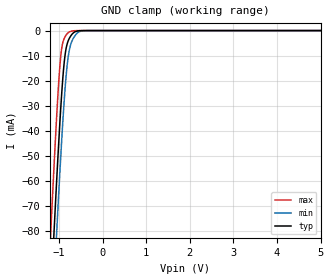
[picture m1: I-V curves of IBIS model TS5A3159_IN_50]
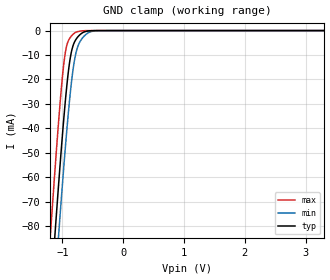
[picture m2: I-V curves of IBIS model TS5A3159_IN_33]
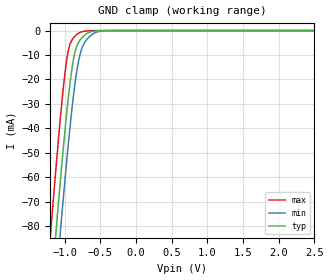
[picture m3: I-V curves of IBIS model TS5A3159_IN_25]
| TEXAS INSTRUMENTS INCORPORATED
| Standard Linear and Logic Group
| IBIS Model of TS5A3159
| 1-OHM SPDT ANALOG SWITCH
| This file contains package information for the following:
|  SOT 6-pin (DBV) package as [Component] TS5A3159_DBV
| This device can be powered at the following Vccs:
|  5 volt Vcc
|  3.3 volt Vcc
|  2.5 volt Vcc
|  1.8 volt Vcc
| This file provides unique models under the [Model Selector] for each Vcc.
| For operation at a specific Vcc, select the appropriate model after each
| [Model Selector] keyword.
[IBIS Ver]   3.2
[Comment char]  |_char
[File Name]   ts5a3159.ibs
[File Rev]   1.1 | a_die
[Date]   January 6, 2009
[Source]   Data created from TI-SPICE simulations at TI-SLL.
[Notes]   The following is an IBIS list for the TS5A3159.
   Please contact sllibis@ti.com with questions and
   comments concerning SLL IBIS models.
   - FILE REV HISTORY
   - 1.1 Release IBIS file on 01/08/09.
   - Power clamp data deleted was deleted as there is no
   power-clamp diode.
   - Non-monotonic data due to FET characteristics.
[Disclaimer] Property of Texas Instruments Incorporated.  Unauthorized
   reproduction and/or distribution is strictly prohibited.
   This product is protected under copyright law.
   Created  2009, (C) Copyright  2009, Texas Instruments
   Incorporated, All Rights Reserved
   UNLESS THERE IS A SIGNED, WRITTEN AGREEMENT TO THE
   CONTRARY, TEXAS INSTRUMENTS (TI) IS PROVIDING THE IBIS
   MODELS  AND WITHOUT ANY WARRANTY, EXPRESSED OR
   IMPLIED.  TI assumes no liability for:
   1) the accuracy of the IBIS models provided to your
   company;
   2) the proper functioning of these IBIS Models in your
   design or for any resulting applications; or
   3) infringement of patents, copyrights or intellectual
   property rights resulting from your use of these IBIS
   models.
   TI provides IBIS Models as a service to our customers.
   You and your company shall not distribute, sell or give
   these models to anyone else without prior written
   permission from TI.
   TI reserves the right to make changes to our products or
   to discontinue any semiconductor product or service
   without notice, and advises our customers to obtain the
   latest version of relevant information to verify, before
   placing orders, that the information being relied on is
   current.
   Please be aware that your receipt and use of the IBIS
   information provided shall serve as acceptance of these
   terms and conditions.  If you do not accept these terms,
   you should return or destroy the IBIS models and any
   other accompanying information immediately.
| Component TS5A3159_DBV 6-PIN SOT
[Component]   TS5A3159_DBV
[Manufacturer]   Texas Instruments, Inc.
[Package]
|   typ   min   max
R_pkg   2.500e-02   1.900e-02   3.700e-02
L_pkg   1.524e-09   1.260e-09   1.751e-09
C_pkg   2.450e-13   1.980e-13   2.640e-13
[Pin]   signal_name   model_name   R_pin   L_pin   C_pin
1   NO   TS5A3159_NX   2.100e-02   1.405e-09   2.460e-13
2   GND   GND   3.700e-02   1.751e-09   2.630e-13
3   NC   TS5A3159_NX   2.600e-02   1.493e-09   2.470e-13
4   COM   TS5A3159_COM   1.900e-02   1.620e-09   2.640e-13
5   VP   POWER   2.400e-02   1.260e-09   1.980e-13
6   IN   TS5A3159_IN   2.100e-02   1.617e-09   2.500e-13
[Series Switch Groups]
| Function Group States
On  1 /   | NO->COM IN HIGH
   | COM->NO IN HIGH
On  2 /   | NC->COM IN LOW
   | COM->NC IN LOW
On  1 /   | IN HIGH
[Series Pin Mapping]   pin_2   model_name   function_table_group
1   4   TS5A3159_NX_S   1
4   1   TS5A3159_COM_S   1
3   4   TS5A3159_NX_S   2
4   3   TS5A3159_COM_S   2
| Model TS5A3159_IN
[Model Selector]   TS5A3159_IN
TS5A3159_IN_50   5 volt Vcc
TS5A3159_IN_33   3.3 volt Vcc
TS5A3159_IN_25   2.5 volt Vcc
TS5A3159_IN_18   1.8 volt Vcc
| Model TS5A3159_NX
[Model Selector]   TS5A3159_NX
TS5A3159_NX_50   5 volt Vcc
TS5A3159_NX_33   3.3 volt Vcc
TS5A3159_NX_25   2.5 volt Vcc
TS5A3159_NX_18   1.8 volt Vcc
| Model TS5A3159_NX_S
[Model Selector]   TS5A3159_NX_S
TS5A3159_NX_50_S   5 volt Vcc
TS5A3159_NX_33_S   3.3 volt Vcc
TS5A3159_NX_25_S   2.5 volt Vcc
TS5A3159_NX_18_S   1.8 volt Vcc
| Model TS5A3159_COM
[Model Selector]   TS5A3159_COM
TS5A3159_COM_50   5 volt Vcc
TS5A3159_COM_33   3.3 volt Vcc
TS5A3159_COM_25   2.5 volt Vcc
TS5A3159_COM_18   1.8 volt Vcc
| Model TS5A3159_COM_S
[Model Selector]   TS5A3159_COM_S
TS5A3159_COM_50_S   5 volt Vcc
TS5A3159_COM_33_S   3.3 volt Vcc
TS5A3159_COM_25_S   2.5 volt Vcc
TS5A3159_COM_18_S   1.8 volt Vcc
[Model]   TS5A3159_NX_50_S
Model_type  Series_switch
| variable   typ   min   max
C_comp   0   0   0
[Temperature Range]   40   100   -40
| Ambient temperature   25   85   -40
[Voltage range]   5   4.5   5.5
[On]
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[Off]
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[Model]   TS5A3159_NX_33_S
Model_type  Series_switch
| variable   typ   min   max
C_comp   0   0   0
[Temperature Range]   40   100   -40
| Ambient temperature   25   85   -40
[Voltage range]   3.3   3   3.6
[On]
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[Off]
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[Model]   TS5A3159_NX_25_S
Model_type  Series_switch
| variable   typ   min   max
C_comp   0   0   0
[Temperature Range]   40   100   -40
| Ambient temperature   25   85   -40
[Voltage range]   2.5   2.3   2.7
[On]
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[Off]
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[Model]   TS5A3159_NX_18_S
Model_type  Series_switch
| variable   typ   min   max
C_comp   0   0   0
[Temperature Range]   40   100   -40
| Ambient temperature   25   85   -40
[Voltage range]   1.8   1.65   1.95
[On]
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[Off]
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[Model]   TS5A3159_COM_50_S
Model_type  Series_switch
| variable   typ   min   max
C_comp   0   0   0
[Temperature Range]   40   100   -40
| Ambient temperature   25   85   -40
[Voltage range]   5   4.5   5.5
[On]
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[Off]
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[Model]   TS5A3159_COM_33_S
Model_type  Series_switch
| variable   typ   min   max
C_comp   0   0   0
[Temperature Range]   40   100   -40
| Ambient temperature   25   85   -40
[Voltage range]   3.3   3   3.6
[On]
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[Off]
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[Model]   TS5A3159_COM_25_S
Model_type  Series_switch
| variable   typ   min   max
C_comp   0   0   0
[Temperature Range]   40   100   -40
| Ambient temperature   25   85   -40
[Voltage range]   2.5   2.3   2.7
[On]
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[Off]
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[Model]   TS5A3159_COM_18_S
Model_type  Series_switch
| variable   typ   min   max
C_comp   0   0   0
[Temperature Range]   40   100   -40
| Ambient temperature   25   85   -40
[Voltage range]   1.8   1.65   1.95
[On]
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[Off]
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| Models and submodels in the file (20): TS5A3159_IN_50 (Input), TS5A3159_IN_33 (Input), TS5A3159_IN_25 (Input), TS5A3159_IN_18 (Input), TS5A3159_NX_50_S (Series_switch), TS5A3159_NX_50 (Terminator), TS5A3159_NX_33_S (Series_switch), TS5A3159_NX_33 (Terminator), TS5A3159_NX_25_S (Series_switch), TS5A3159_NX_25 (Terminator), TS5A3159_NX_18_S (Series_switch), TS5A3159_NX_18 (Terminator), TS5A3159_COM_50_S (Series_switch), TS5A3159_COM_50 (Terminator), TS5A3159_COM_33_S (Series_switch), TS5A3159_COM_33 (Terminator), TS5A3159_COM_25_S (Series_switch), TS5A3159_COM_25 (Terminator), TS5A3159_COM_18_S (Series_switch), TS5A3159_COM_18 (Terminator)
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[Model]   TS5A3159_IN_50
Model_type  Input
Vinl=0.8
Vinh=2.4
| variable   typ   min   max
C_comp   1.80pF   1.37pF   2.42pF
[Temperature Range]   40   100   -40
| Ambient temperature   25   85   -40
[Voltage range]   5   4.5   5.5
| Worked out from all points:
|   GND clamp passes 1 mA (typ) near -0.68 V on its own axis
[GND Clamp]
| TS5A3159_IN_50
|   Voltage   I(typ)   I(min)   I(max)
-5V       -1.6A      -1.615A    -1.582A
-1.21V    -114.4mA   -135.5mA   -88mA
-1.185V   -105.4mA   -126.5mA   -78.99mA
-1.105V   -77.24mA   -98.26mA   -51.05mA
-1.055V   -60.34mA   -81.11mA   -34.72mA
-960mV    -31.01mA   -50.33mA   -10.28mA
-860mV    -9.673mA   -23.05mA   -2.449mA
-805mV    -4.875mA   -12.64mA   -1.097mA
-755mV    -2.838mA   -7.118mA   -471.6uA
-640mV    -543.8uA   -2.191mA   -50.87uA
-450mV    -10.31uA   -96.88uA   -94.69nA
5V        94.34pA    6.928nA    60pA
[Model]   TS5A3159_IN_33
Model_type  Input
Vinl=0.6
Vinh=2.0
| variable   typ   min   max
C_comp   1.87pF   1.46pF   2.37pF
[Temperature Range]   40   100   -40
| Ambient temperature   25   85   -40
[Voltage range]   3.3   3   3.6
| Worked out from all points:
|   GND clamp passes 1 mA (typ) near -0.68 V on its own axis
[GND Clamp]
| TS5A3159_IN_33
|   Voltage   I(typ)   I(min)   I(max)
-3.3V     -925.1mA   -942.5mA   -904.5mA
-1.2V     -110.8mA   -131.9mA   -84.38mA
-1.18V    -103.6mA   -124.7mA   -77.2mA
-1.115V   -80.69mA   -101.7mA   -54.44mA
-1.06V    -62mA      -82.81mA   -36.29mA
-970mV    -33.84mA   -53.42mA   -12.12mA
-930mV    -23.12mA   -41.38mA   -6.239mA
-875mV    -11.83mA   -26.59mA   -2.952mA
-785mV    -3.919mA   -10.01mA   -780.9uA
-670mV    -903.5uA   -3.024mA   -102.5uA
-475mV    -19.29uA   -157.5uA   -251.4nA
3.3V      59.38pA    3.794nA    39.6pA
[Model]   TS5A3159_IN_25
Model_type  Input
Vinl=0.6
Vinh=1.8
| variable   typ   min   max
C_comp   1.92pF   1.53pF   2.35pF
[Temperature Range]   40   100   -40
| Ambient temperature   25   85   -40
[Voltage range]   2.5   2.3   2.7
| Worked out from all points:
|   GND clamp passes 1 mA (typ) near -0.68 V on its own axis
[GND Clamp]
| TS5A3159_IN_25
|   Voltage   I(typ)   I(min)   I(max)
-2.5V     -609.8mA   -628.5mA   -587.4mA
-1.2V     -110.8mA   -131.9mA   -84.38mA
-1.18V    -103.6mA   -124.7mA   -77.2mA
-1.12V    -82.43mA   -103.5mA   -56.15mA
-1.055V   -60.34mA   -81.11mA   -34.72mA
-1V       -42.75mA   -62.93mA   -18.92mA
-960mV    -31.01mA   -50.33mA   -10.28mA
-880mV    -12.64mA   -27.82mA   -3.14mA
-800mV    -4.611mA   -11.93mA   -1.009mA
-700mV    -1.431mA   -4.068mA   -186.6uA
-480mV    -21.8uA    -173.1uA   -304.3nA
2.5V      44.7pA     2.773nA    30pA
